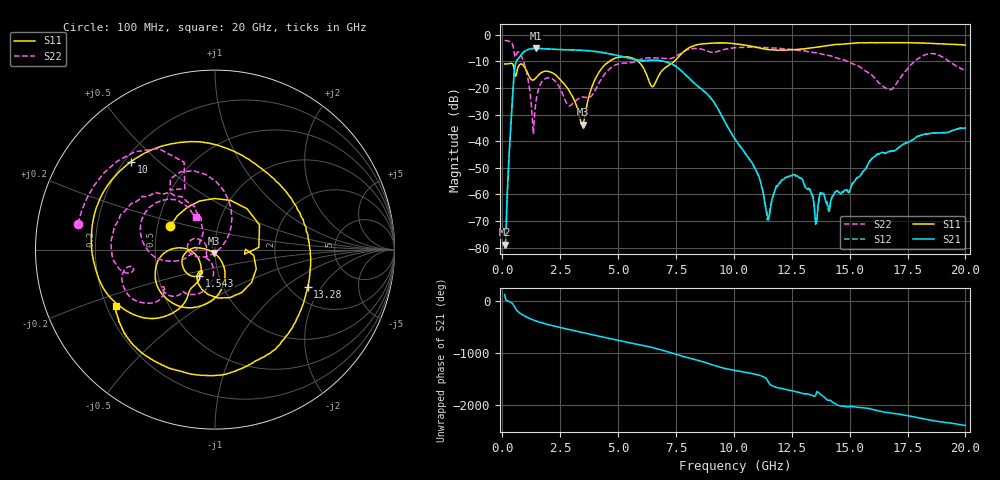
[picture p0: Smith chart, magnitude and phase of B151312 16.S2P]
!  2-Port S-parameters saved by WinCal
! VAR MeasName=S-Parameters (CALIBRATED_DATA) read from VNA (N5244A)
! VAR MeasDate=12/8/2015 5:44:44 PM
! VAR NAME=B151312 16
! VAR FILENAME=B151312 16.S2P
! VAR DATE=12/8/2015 5:44:44 PM
! VAR PHYS_PORTS=1,2
# Hz S DB R 50
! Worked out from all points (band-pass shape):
!   401 points, 100 MHz to 20 GHz, reference 50 ohm
!   highest |S21| = -5.18 dB at 1.443 GHz (marker M1); lowest = -78.9 dB at 100 MHz (marker M2)
!   |S21| within 3 dB of the highest: 759.6 MHz to 5.165 GHz (4.406 GHz wide, 149 % of centre)
!   lowest |S11| = -33.8 dB at 3.483 GHz (marker M3), VSWR 1.04, Z = 49.4 - j1.92 ohm
!   |S11| at or under -10 dB: start of sweep to 4.626 GHz; 5.859 GHz to 7.429 GHz (1.569 GHz wide, 23.6 % of centre)
!   |S22| runs from -37.3 to -2.2 dB; largest |S21 - S12| = 0.0015
!   S11 on the Smith chart (normalised r, x): 100 MHz: 0.58, +0.16; 1.543 GHz: 0.81, -0.24; 10 GHz: 0.23, +0.41; 13.28 GHz: 2.48, -1.50; 20 GHz: 0.24, -0.25
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1e8  -11.00 152.6  -78.88 115.9  -79.39 120.8  -2.19 169.3
4.4825e8  -10.95 28.9  -22.66 -62.2  -22.67 -62.2  -3.80 119.2
5.975e8  -15.39 0.7  -10.08 -169.6  -10.08 -169.6  -7.61 127.0
9.4575e8  -11.92 -98.5  -6.39 69.6  -6.39 69.6  -10.84 74.9
1.44325e9  -16.34 -118.5  -5.18 -27.2  -5.18 -27.1  -25.80 -136.8
1.54275e9  -15.39 -121.2  -5.19 -41.9  -5.19 -41.9  -21.19 -151.1
2.53775e9  -17.22 179.4  -5.61 -157.6  -5.61 -157.7  -20.97 146.5
3.43325e9  -33.76 -133.2  -5.90 112.8  -5.90 112.8  -23.44 -143.2
3.483e9  -33.83 -107.5  -5.92 107.9  -5.92 107.9  -23.43 -140.8
4.677e9  -9.71 -105.0  -7.28 -9.0  -7.27 -9.0  -12.55 -105.0
5.5725e9  -8.68 -154.7  -9.06 -93.3  -9.07 -93.4  -10.49 -127.7
6.7665e9  -15.20 -118.6  -9.68 149.3  -9.69 149.3  -8.77 -144.4
8.06e9  -4.96 -138.7  -16.31 -17.4  -16.31 -17.5  -5.50 -148.2
1.000025e10  -3.39 133.6  -38.57 108.8  -38.60 108.6  -4.95 -173.3
1.005e10  -3.43 131.3  -39.19 104.9  -39.25 104.8  -4.90 -174.0
1.1443e10  -5.55 64.8  -67.07 -81.0  -69.48 -77.2  -4.93 165.2
1.228875e10  -5.76 23.6  -53.62 97.3  -53.46 97.9  -5.41 152.7
1.328375e10  -5.09 -22.0  -57.94 0.4  -58.43 -3.8  -6.56 140.0
1.338325e10  -4.99 -25.7  -60.35 -11.9  -60.05 -12.7  -6.67 138.0
1.67165e10  -3.02 -113.7  -43.91 12.4  -43.72 11.7  -20.68 161.0
1.835825e10  -3.25 -136.0  -37.29 -114.9  -37.29 -114.9  -7.32 165.0
2e10  -3.94 -150.4  -35.15 132.9  -35.17 131.6  -13.53 119.8
